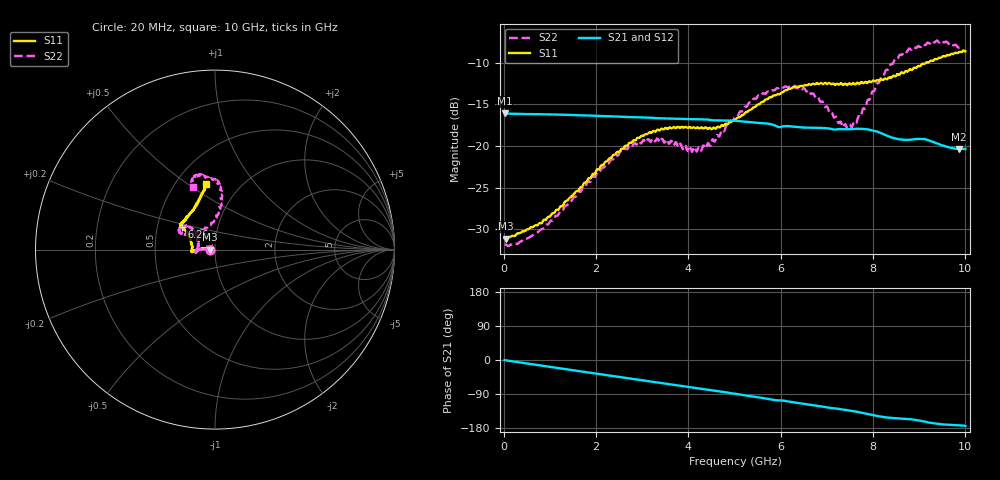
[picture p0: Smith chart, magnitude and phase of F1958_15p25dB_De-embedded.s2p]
! Integrated Device Technology
! Corporate Headquarters
! 6024 Silver Creek Valley Road
! San Jose, CA 95138  USA
! Phone:  1-408-284-8200
! Toll Free:  1-800-223-1366
! Webpage:  http://www.idt.com/
! Timing and RF Division
! 515 Groton Road, Suite 102
! Westford, MA 01886-6024
! Device:  F1958
! Description: 7-bit 0.25 dB Digital Step Attenuator
! Frequency:  0.001 -  6.000 GHz
! Package:  4x4 mm Thin QFN Plastic Package: 24 pin
! Ports:  2 RF, 12 DC
!  Pin  1  = D0
!  Pin  2  = VDD
!  Pin  3  = VMODE
!  Pin  4  = GND
!  Pin  5  = RF1  =  Port 1
!  Pin  6  = GND
!  Pin  7  = GND
!  Pin  8  = GND
!  Pin  9  = GND
!  Pin 10  = GND
!  Pin 11  = GND
!  Pin 12  = GND
!  Pin 13  = GND
!  Pin 14  = RF2  =  Port 2
!  Pin 15  = GND
!  Pin 16  = LE
!  Pin 17  = CLK
!  Pin 18  = DATA
!  Pin 19  = D6
!  Pin 20  = D5
!  Pin 21  = D4
!  Pin 22  = D3
!  Pin 23  = D2
!  Pin 24  = D1
! State:  61
! Atten State:  15.25 dB
! Voltage:  +3.30 Volts
! Current:  0.258 mA
! Data:  The device was measured on a F1958 evaluation board which has
!  individual transmission lines to the RF pins.  Data was collected
!  using a calibrated network analyzer.  The evaluation board was
!  de-embedded using Automatic Fixture Removal (AFR).
!  The reference plane is the edge of the package pin.
! Misc:
!  Action Tracker AT0419
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# GHz S dB R 50
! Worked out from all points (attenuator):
!   500 points, 20 MHz to 10 GHz, reference 50 ohm
!   highest |S21| = -16.08 dB at 20 MHz (marker M1); lowest = -20.4 dB at 9.86 GHz (marker M2)
!   lowest |S11| = -31.1 dB at 40 MHz (marker M3), VSWR 1.06, Z = 47.3 - j0.0664 ohm
!   |S11| at or under -10 dB: start of sweep to 9.144 GHz
!   |S22| runs from -32.0 to -7.3 dB; largest |S21 - S12| = 0.00057
!   S11 on the Smith chart (normalised r, x): 20 MHz: 0.95, -0.00; 6.26 GHz: 0.67, +0.18; 10 GHz: 0.69, +0.59
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0.02  -31.07 -178.5  -16.08 -0.5  -16.08 -0.5  -31.86 -178.6
0.04  -31.10 -178.6  -16.09 -0.9  -16.09 -0.8  -31.81 -177.8
0.32  -30.48 177.0  -16.13 -5.9  -16.13 -5.9  -31.68 177.6
0.84  -29.10 174.8  -16.18 -15.2  -16.17 -15.2  -29.96 177.7
1.7  -24.86 175.6  -16.31 -30.5  -16.30 -30.5  -25.09 176.6
2.6  -20.23 179.8  -16.49 -46.4  -16.47 -46.4  -20.50 -178.3
2.92  -19.01 -177.3  -16.54 -52.1  -16.53 -52.2  -19.42 -174.9
3.36  -18.10 -174.7  -16.65 -59.9  -16.65 -60.0  -19.37 -170.7
4.24  -17.90 -179.8  -16.79 -75.3  -16.80 -75.3  -20.14 167.2
4.5  -17.98 174.3  -16.89 -80.2  -16.90 -80.2  -19.53 151.8
5.02  -16.84 159.8  -16.96 -89.3  -16.97 -89.3  -16.38 138.6
5.54  -14.96 149.8  -17.22 -98.9  -17.22 -98.9  -13.94 140.0
6.26  -12.97 146.1  -17.65 -111.5  -17.67 -111.5  -12.97 150.9
6.68  -12.55 144.2  -17.79 -118.6  -17.80 -118.6  -13.72 153.3
7.3  -12.46 138.1  -17.96 -129.9  -17.96 -129.7  -17.05 132.5
7.5  -12.51 135.4  -17.98 -133.5  -17.98 -133.5  -17.41 114.4
7.68  -12.47 132.5  -17.92 -137.3  -17.91 -137.3  -16.44 97.6
8.34  -11.76 116.7  -18.84 -152.3  -18.84 -152.4  -10.68 82.4
8.7  -10.98 110.2  -19.26 -155.4  -19.25 -155.3  -8.63 87.9
9.26  -9.72 102.4  -19.43 -166.1  -19.43 -166.1  -7.49 99.6
9.86  -8.72 98.0  -20.37 -172.5  -20.39 -172.3  -8.17 108.7
10  -8.60 98.1  -20.32 -173.9  -20.37 -173.7  -8.69 109.5
